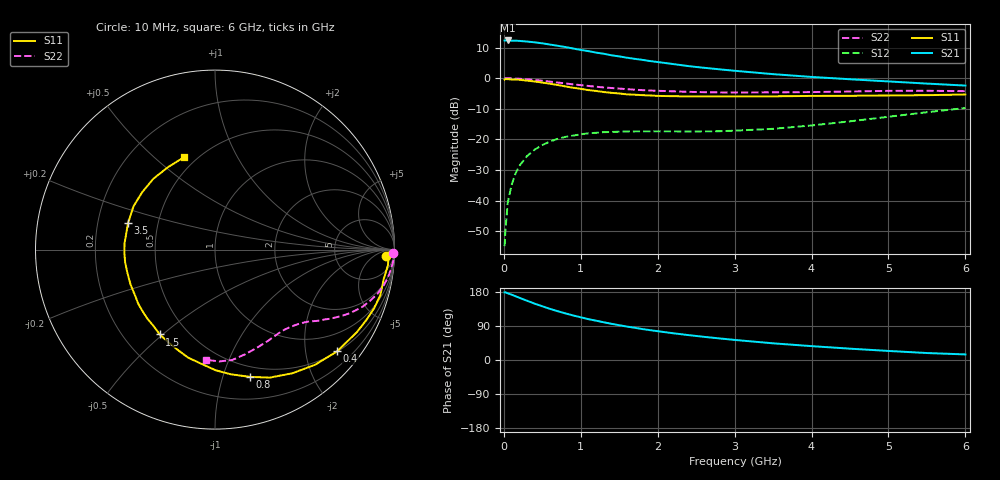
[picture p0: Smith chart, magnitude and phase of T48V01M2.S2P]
! Infineon Technologies  Discrete & RF Semiconductors
! BFR182T
! Si NPN RF Bipolar Junction Transistor in SC75
! VCE = 8 V  IC = 1.2 mA
! Common Emitter S-Parameters:  October  1999
# GHz  S  MA  R  50
!  f  S11  S21  S12  S22
! GHz  MAG  ANG  MAG  ANG  MAG  ANG  MAG  ANG
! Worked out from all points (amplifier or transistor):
!   36 points, 10 MHz to 6 GHz, reference 50 ohm
!   highest |S21| = 12.4 dB at 50 MHz (marker M1)
!   |S21| within 3 dB of that: start of sweep to 978 MHz
!   unconditionally stable (mu >= 1): 2.351 GHz to 4.568 GHz
!   at 250 MHz: K = 0.10, MSG = 19.6 dB, |S12| = -27.1 dB
!   at 1.4 GHz: K = 0.61, MSG = 12.5 dB, |S12| = -17.6 dB
!   at 6 GHz: K = 0.83, MSG = 3.7 dB, |S12| = -9.7 dB
!   S11 on the Smith chart (normalised r, x): 10 MHz: 26, -20; 400 MHz: 0.51, -2.68; 800 MHz: 0.40, -1.23; 1.5 GHz: 0.35, -0.49; 3.5 GHz: 0.33, +0.13; 6 GHz: 0.43, +0.63
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0.01  0.9536 -2.1  4.126 178.6  0.0018 73.1  0.9904 -1.2
0.02  0.9696 -0.8  4.146 178.8  0.0032 96.6  0.9999 -0.8
0.05  0.9675 -5.2  4.147 176.1  0.0091 88.8  0.9957 -2.1
0.1  0.9543 -9.9  4.112 172.5  0.018 83.5  0.9943 -4.1
0.15  0.9557 -15.5  4.115 168.3  0.0273 81.7  0.987 -6.1
0.2  0.9446 -20.3  4.079 164.3  0.0368 79.0  0.9804 -8.0
0.3  0.9148 -30.1  3.98 156.5  0.0532 73.1  0.9622 -11.7
0.4  0.8855 -39.8  3.865 148.7  0.068 67.2  0.9376 -15.3
0.5  0.8502 -49.0  3.721 141.8  0.0809 62.5  0.9095 -18.3
0.6  0.8126 -58.0  3.555 134.9  0.0925 57.8  0.8812 -21.2
0.8  0.7356 -74.6  3.239 123.0  0.1102 50.3  0.8224 -25.8
0.9  0.6998 -82.9  3.063 117.6  0.1155 47.3  0.7944 -27.8
1.1  0.6398 -97.1  2.773 107.7  0.126 42.1  0.748 -31.0
1.3  0.595 -110.8  2.51 99.5  0.1315 38.3  0.7079 -33.8
1.5  0.564 -123.1  2.275 91.8  0.134 36.1  0.6783 -36.0
1.8  0.5293 -140.1  1.999 81.7  0.1355 33.8  0.6394 -39.5
2.2  0.5091 -157.5  1.706 70.6  0.1357 34.0  0.6114 -43.7
2.8  0.5053 -178.1  1.4 57.0  0.136 38.7  0.5867 -51.1
3.5  0.5064 163.2  1.167 44.0  0.1491 47.8  0.588 -59.9
4.5  0.5166 141.8  0.963 29.9  0.1977 57.6  0.6068 -73.9
5.5  0.5289 119.5  0.818 18.4  0.2786 59.2  0.6237 -87.9
6  0.5424 108.7  0.759 14.7  0.3264 56.8  0.6158 -94.5
